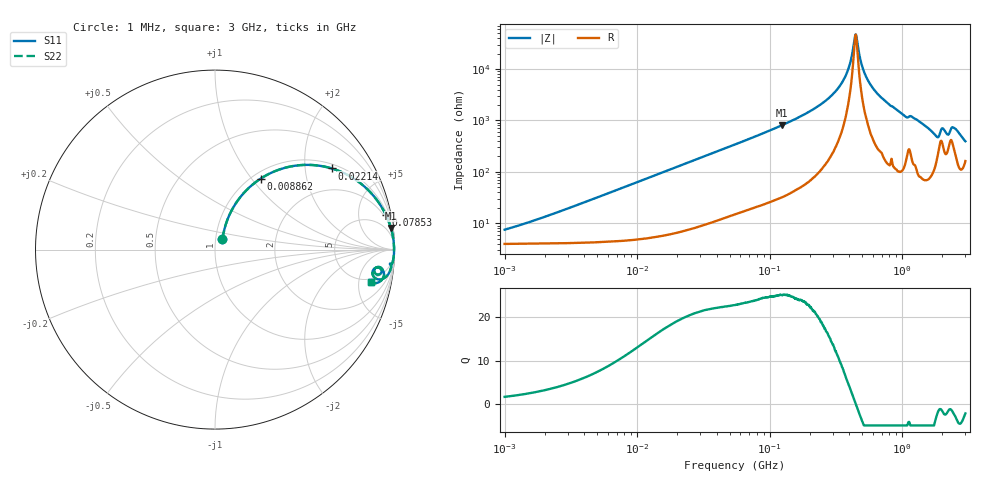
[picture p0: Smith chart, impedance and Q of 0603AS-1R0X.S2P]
!s-Parameter Generated by FASTRON Sdn. Bhd.
!FASTRON P/N : 0603AS-1R0X
!Keysight Technologies: E4991B_MY54100416_A.01.15
!Date created: Tue Oct 17 14:40:26 2023
!Version  : Rev01 Tue Oct 17 14:40:26 2023
!Data & Calibration Information:
!Freq	S11	S21	S12	S22
!PortZ  Port1:50+j0  Port2:50+j0
!When reading reference impedance value at option line is always used.
! Remarks : This data is being provided solely for informational purposes.
# Hz S dB R 50
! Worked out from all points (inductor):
!   1601 points, 1 MHz to 3 GHz, reference 50 ohm
!   read as one part in series: L = 1.01 uH near 1.917 MHz
!   highest Q = 25.2 at 123.8 MHz (marker M1), where L = 1.04 uH
!   self-resonance near 445.8 MHz
!   S11 on the Smith chart (normalised r, x): 1 MHz: 1.08, +0.13; 8.862 MHz: 1.09, +1.11; 22.14 MHz: 1.14, +2.77; 78.53 MHz: 1.41, +9.83; 3 GHz: 4.24, -7.17
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1000000  -22.85 54.6  -0.35 -3.5  -0.35 -3.5  -22.85 54.6
3804036  -12.84 67.2  -0.58 -13.0  -0.58 -13.0  -12.84 67.2
8861669  -6.53 57.2  -1.48 -28.0  -1.48 -28.0  -6.53 57.2
1.447069e7  -3.70 45.8  -2.87 -40.7  -2.87 -40.7  -3.70 45.8
2.214172e7  -2.03 34.8  -4.85 -52.3  -4.85 -52.3  -2.03 34.8
5.477226e7  -0.46 16.1  -11.11 -71.3  -11.11 -71.3  -0.46 16.1
7.852918e7  -0.25 11.4  -14.09 -76.2  -14.09 -76.2  -0.25 11.4
1.238204e8  -0.11 7.0  -18.24 -80.7  -18.24 -80.7  -0.11 7.0
2.083556e8  -0.04 3.6  -24.06 -83.8  -24.06 -83.8  -0.04 3.6
2.827291e8  -0.03 2.0  -28.97 -84.3  -28.97 -84.3  -0.03 2.0
3.48855e8  -0.02 1.1  -34.47 -82.5  -34.47 -82.5  -0.02 1.1
3.933705e8  -0.02 0.5  -40.20 -76.9  -40.20 -76.9  -0.02 0.5
4.457915e8  -0.02 0.0  -53.47 -1.9  -53.47 -1.9  -0.02 0.0
4.593788e8  -0.02 -0.1  -50.27 46.3  -50.27 46.3  -0.02 -0.1
5.001674e8  -0.02 -0.5  -40.89 75.7  -40.89 75.7  -0.02 -0.5
5.473095e8  -0.02 -0.9  -35.96 81.0  -35.96 81.0  -0.02 -0.9
7.925923e8  -0.04 -2.7  -26.40 83.5  -26.40 83.5  -0.04 -2.7
1.800756e9  -0.64 -10.3  -14.55 62.6  -14.55 62.6  -0.64 -10.3
2.000286e9  -0.69 -6.4  -17.62 51.5  -17.62 51.5  -0.69 -6.4
2.199798e9  -0.83 -8.7  -15.36 53.5  -15.36 53.5  -0.83 -8.7
2.431346e9  -0.55 -6.7  -17.83 58.1  -17.83 58.1  -0.55 -6.7
3e9  -1.05 -11.8  -12.95 53.8  -12.95 53.8  -1.05 -11.8
